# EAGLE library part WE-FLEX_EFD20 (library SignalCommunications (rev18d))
WE-FLEX Flexible Transformer for DC/DC Converter Characteristics Transformer with 6 identical windings 4 sizes with 5 different lengths of air gap each Insulation test voltage 500 VAC Low leakage inductance Operating temperature: –40 ºC to +125 ºC By using different circuits more than 375 transformer solutions and about 125 choke solutions possible. Consequently, quick prototyping possibilities Applications All kind of switching regulators -Flyback converters -Forward converters -Push-pull converters -Step-up/step-down converters -SEPIC converter Details see: http://katalog.we-online.de/en/pbs/WE-FLEX? Updated by Dan Xu 2014-07-07 2014 (C) Wurth Elektronik
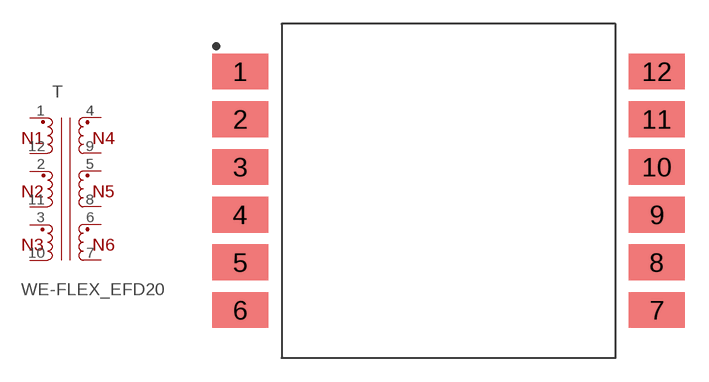
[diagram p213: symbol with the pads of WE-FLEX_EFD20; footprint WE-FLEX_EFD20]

Designator prefix T

## WE-FLEX_EFD20_749196500, WE-FLEX_EFD20_749196501, WE-FLEX_EFD20_749196510, WE-FLEX_EFD20_749196511, WE-FLEX_EFD20_749196520, WE-FLEX_EFD20_749196521, WE-FLEX_EFD20_749196530, WE-FLEX_EFD20_749196531, WE-FLEX_EFD20_749196540, WE-FLEX_EFD20_749196541  [WE-FLEX_EFD20]
1  1  pas
2  11  pas
3  9  pas
4  2  pas
5  4  pas
6  6  pas
7  7  pas
8  5  pas
9  3  pas
10  8  pas
11  10  pas
12  12  pas

## Footprint WE-FLEX_EFD20 (pad centres in mm)
smd 3.5 x 2.25: 1 -13.1,7.5; 2 -13.1,4.5; 3 -13.1,1.5; 4 -13.1,-1.5; 5 -13.1,-4.5; 6 -13.1,-7.5; 7 13.1,-7.5; 8 13.1,-4.5; 9 13.1,-1.5; 10 13.1,1.5; 11 13.1,4.5; 12 13.1,7.5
